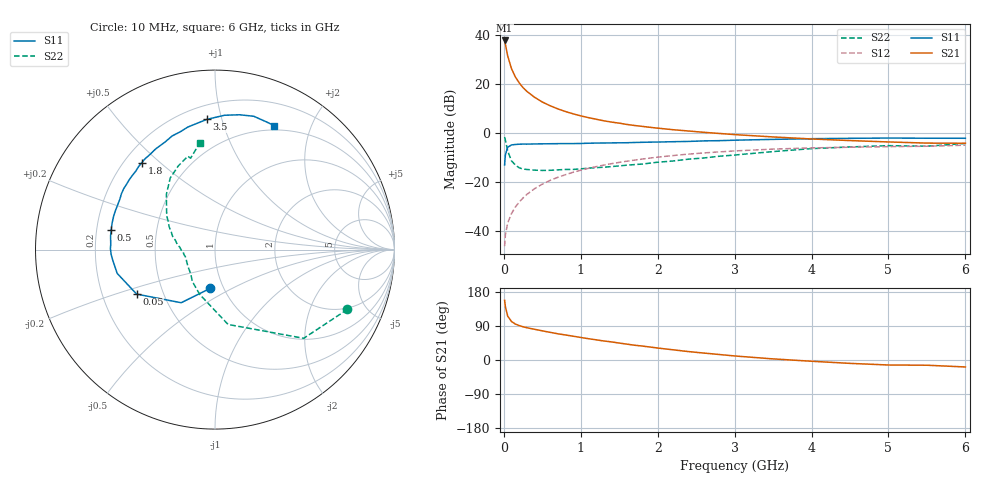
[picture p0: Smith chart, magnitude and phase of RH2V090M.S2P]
! SIEMENS Small Signal Semiconductors
! BFR106
! Si NPN RF Bipolar Junction Transistor in SOT23
! VCE = 2 V  IC = 90 mA
! Common Emitter S-Parameters:  August  1996
# GHz  S  MA  R  50
!  f  S11  S21  S12  S22
! GHz  MAG  ANG  MAG  ANG  MAG  ANG  MAG  ANG
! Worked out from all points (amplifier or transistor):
!   36 points, 10 MHz to 6 GHz, reference 50 ohm
!   highest |S21| = 37.6 dB at 10 MHz (marker M1)
!   |S21| within 3 dB of that: start of sweep to 29.19 MHz
!   unconditionally stable (mu >= 1): 144.3 MHz to 3.161 GHz; 4.574 GHz to end of sweep
!   at 250 MHz: K = 1.08, MAG = 20.7 dB, |S12| = -26.7 dB
!   at 1.4 GHz: K = 1.08, MAG = 6.7 dB, |S12| = -12.7 dB
!   at 6 GHz: K = 1.02, MAG = -0.4 dB, |S12| = -5.1 dB
!   S11 on the Smith chart (normalised r, x): 10 MHz: 0.87, -0.39; 50 MHz: 0.35, -0.23; 500 MHz: 0.26, +0.09; 1.8 GHz: 0.27, +0.44; 3.5 GHz: 0.29, +0.90; 6 GHz: 0.45, +1.49
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0.01  0.2177 -97.0  76.02 157.6  0.0048 76.2  0.8096 -24.3
0.02  0.351 -122.5  63.75 140.9  0.0081 67.7  0.6989 -45.0
0.05  0.502 -150.4  36.69 115.9  0.0143 60.3  0.4233 -80.1
0.1  0.5607 -166.3  20.12 101.5  0.0223 64.0  0.2641 -108.7
0.15  0.572 -173.7  13.65 94.8  0.0303 69.2  0.2181 -125.4
0.2  0.5791 -177.2  10.36 90.8  0.0382 71.1  0.1908 -135.1
0.25  0.5828 179.4  8.27 87.6  0.0464 72.1  0.1805 -144.2
0.3  0.5816 177.2  6.932 85.2  0.0548 73.2  0.1767 -149.1
0.4  0.5867 172.6  5.247 81.0  0.0718 73.3  0.1711 -157.7
0.5  0.5891 169.1  4.214 76.9  0.0886 72.8  0.1688 -163.0
0.6  0.5921 165.3  3.538 73.1  0.1055 71.8  0.1699 -166.4
0.7  0.5946 161.8  3.057 69.2  0.1219 70.5  0.1734 -169.4
0.9  0.5965 155.7  2.418 62.8  0.155 67.4  0.177 -175.5
1.1  0.6068 149.3  2.018 56.2  0.1865 64.3  0.1883 -179.2
1.4  0.616 141.0  1.637 47.7  0.2319 59.1  0.2022 174.6
1.8  0.6334 130.1  1.339 36.8  0.2882 52.0  0.2281 166.4
2.2  0.6515 120.3  1.145 26.9  0.3399 45.1  0.2631 157.9
2.8  0.6841 106.5  0.96 14.5  0.4037 34.8  0.3288 144.9
3.5  0.7269 93.6  0.815 2.9  0.4603 23.6  0.4097 131.4
4.5  0.7635 79.7  0.687 -8.9  0.5028 9.4  0.5091 113.7
5.5  0.7672 68.3  0.61 -13.8  0.5267 0.8  0.5273 104.9
6  0.7657 64.4  0.606 -18.4  0.5529 -5.9  0.5994 98.2
